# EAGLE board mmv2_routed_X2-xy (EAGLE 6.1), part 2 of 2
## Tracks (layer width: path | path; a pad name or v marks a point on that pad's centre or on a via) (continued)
GLC1P  (via drill 0.5) (continued)
  Top 0.2: R22.1 61.21,31.4 63.21,31.4 R21.1 63.31,31.4 67.31,31.4 | R19.1 73.31,29.5 73.21,29.5 71.31,31.4 R20.1 67.31,31.4 | R26.1 40.81,31.4 R25.1 46.91,31.4 | R23.1 53.01,31.5 51.01,31.5 R24.1 50.91,31.4 46.91,31.4 | 6.41,31.5 10.21,31.5 R32.1 10.31,31.4 12.31,31.4 R31.1 | 6.41,31.5 2.61,31.5 R33.1 | R34.1 25.51,43.2 21.31,43.2 20.41,44.1 D125.A | 21.51,31.4 22.51,31.4 R29.1 22.61,31.3 23.41,30.5 29.61,30.5 29.66,30.45 | 21.51,31.4 R30.1 | R27.1 32.71,31.4 30.71,31.4 R28.1 30.61,31.4 29.66,30.45 | 29.66,30.45 29.51,30.3 29.51,23.8 | 21.51,31.4 v21.51,32.7 | 6.41,23.8 6.41,31.5 | 46.91,23.8 46.91,31.4 | 67.31,23.8 67.31,31.4
  Top 1.676: D65.A D67.C D69.A D71.C 67.31,23.8 D75.C | D75.C D73.A | D75.C D77.A D79.C D83.C | D83.C D81.A | D83.C D85.A D87.C 46.91,23.8 D89.A D91.C D93.A D95.C D97.A D99.C D101.A 29.51,23.8 D103.C D105.A D107.C D109.A D111.C D113.A D115.C D117.A D119.C 6.41,23.8 D121.A D123.C
  Bottom 0.2: v21.51,32.7 21.51,39.9 20.61,40.8 D127.C | D95.C 39.31,22.6 39.31,7.3 38.11,6.1 JP21.2
  Bottom 1.676: D127.C D125.A
  pour Top: 79.51,33 79.51,0.5 0.51,0.5 0.51,33
GLCN
  Top 1.676: JP17.1 JP16.1 JP15.1 JP14.1 JP13.1 JP12.1 JP11.1 JP4.1 JP10.1 JP9.1 JP8.1 JP7.1 JP6.1 JP5.1 JP2.1 JP1.1
  Bottom 0.2: JP18.1 77.51,59.4 78.61,60.5 78.61,96.5 76.51,98.6 68.61,98.6 68.61,96.2 JP17.1
  pour Bottom (isolate 0.254): 79.51,99.5 79.51,55 64.51,55 64.01,95 9.51,95 9.51,99.5
GLCP
  Top 0.2: R10.1 38.01,69.5 35.91,69.5 R9.1 35.81,69.5 27.91,69.5 R8.1 27.81,69.6 25.71,69.6 R7.1 25.61,69.5 R6.1 15.61,69.5 R5.1 15.51,69.6 11.61,69.6 | R1.1 5.41,69.6 7.51,69.6 R2.1 7.61,69.6 11.61,69.6 | R14.1 58.31,69.6 56.21,69.6 R13.1 56.11,69.6 52.21,69.6 | R11.1 48.21,69.5 R12.1 48.31,69.6 52.21,69.6 | 72.51,69.5 R16.1 66.41,69.5 R15.1 | 72.51,69.5 76.41,69.5 R17.1 | R18.1 55.31,57.2 55.91,57.8 60.01,57.8 60.91,56.9 D63.C | 72.51,77.14 72.51,69.5 | 52.21,77.14 52.21,69.6 | 11.61,77.14 11.61,69.6
  Top 1.676: D1.A D3.C D5.A D7.C 11.61,77.14 D9.A D11.C D13.A D15.C D19.C | D19.C D17.A | D19.C D21.A D23.C D27.C | D27.C D25.A | D27.C D29.A D31.C D35.C | D35.C D33.A | D35.C D37.A D39.C 52.21,77.14 D43.C | D43.C D41.A | D43.C D45.A D47.C D51.C | D51.C D49.A | D59.C D57.A 72.51,77.14 D53.A | D53.A D55.C | D53.A D51.C
  Bottom 0.2: D47.C 61.91,76.2 61.91,60.7 61.31,60.1 D61.A | JP4.2 42.01,93.6 42.01,78.3 43.11,77.2 D33.A
  Bottom 1.676: D63.C D61.A
  pour Top (isolate 0.254): 79.51,99.5 79.51,68 0.51,68 0.51,99.5
GND  (via drill 0.5)  (1 unrouted)
  Top 0.2: OK1.3 2.61,65.8 3.51,66.7 9.21,66.7 10.11,65.8 OK2.3 10.21,65.7 OK3.3 12.71,65.8 13.61,66.7 19.41,66.7 20.31,65.8 OK4.3 20.41,65.7 22.81,65.7 OK5.3 22.91,65.8 23.81,66.7 29.51,66.7 30.41,65.8 OK6.3 30.51,65.7 33.01,65.7 OK7.3 33.11,65.8 34.01,66.7 39.71,66.7 40.61,65.8 OK8.3 40.71,65.7 43.11,65.7 OK9.3 | 25.41,35.3 OK27.3 25.41,35.2 24.51,34.3 18.71,34.3 17.81,35.2 OK28.3 17.71,35.3 15.31,35.3 OK29.3 15.21,35.2 14.31,34.3 8.61,34.3 7.71,35.2 OK30.3 7.61,35.3 5.11,35.3 OK31.3 | 34.21,53.8 U1.18 34.26,53.8 | X2.5 11.91,52.4 JP3.5 22.71,52.4 23.71,53.4 25.01,53.4 26.01,54.4 32.41,54.4 33.01,53.8 34.26,53.8 | OK10.3 53.31,65.7 OK11.3 | v47.81,53.6 47.41,53.8 45.71,53.8 U1.63 45.61,53.8 44.81,53.8 44.51,53.5 41.41,53.5 41.31,53.6 40.61,53.6 40.51,53.55 40.26,53.3 v38.51,53.3 | OK25.3 35.61,35.3 38.11,35.3 OK24.3 | v38.51,54.9 38.21,54.9 38.21,56.2 U1.12 | U1.31 34.31,47.3 35.71,47.3 v35.91,47.5 | OK19.3 66.11,35.3 68.51,35.3 OK18.3 68.61,35.2 69.51,34.3 75.31,34.3 76.21,35.2 OK17.3 | v70.61,46 70.31,45.7 68.21,45.7 X1.3 | OK14.3 71.21,65.7 73.61,65.7 OK15.3 | OK23.3 45.81,35.3 48.21,35.3 OK22.3 | v45.61,43.6 43.57,43.6 43.21,43.95 43.21,44.9 U1.47 | OK20.3 58.41,35.3 55.91,35.3 OK21.3 | OK12.3 61.01,65.7 OK13.3 | S1.4 56.71,49.7 60.41,49.7 61.51,48.6 C2.- 61.61,48.5 61.91,48.2 68.11,48.2 X1.5 | 34.26,53.8 35.01,53.8 35.71,54.5 v35.71,54.6
  Top 1.016: X2.3 2.62,55.01 1.91,54.3
  Bottom 0.2: X2.5 11.91,52.5 11.91,55 X2.3 11.91,55.1 12.91,56.1 12.91,65.5 OK3.3 | 25.41,35.3 25.11,35.6 25.11,46 23.61,47.5 23.61,51.5 22.71,52.4 JP3.5 | 25.41,35.3 OK27.3 | v47.81,53.6 49.51,56.3 49.51,56.8 OK16.3 49.61,56.9 50.51,57.8 50.51,65.4 OK10.3 | C5.2 38.91,56.3 38.91,55.3 v38.51,54.9 38.21,54.6 38.21,54.1 | C6.2 35.51,48.1 35.51,47.7 v35.91,47.5 36.31,47.1 36.31,36 35.61,35.3 OK25.3 35.61,35.2 35.71,35.1 35.71,32.8 37.01,31.5 44.41,31.5 45.41,32.5 45.41,34.9 45.71,35.2 OK23.3 45.71,35.3 45.61,35.4 v45.61,43.6 C9.2 | 38.21,53.3 38.21,52.5 34.71,49 C6.2 | 38.21,53.3 38.21,54.1 | 31.11,48 31.01,44.9 31.71,44.2 OK32.3 | 34.41,49.1 C6.2 | 38.21,53.3 v38.51,53.3 | C4.2 78.31,42.8 77.91,42.4 77.91,37 76.21,35.3 OK17.3 | v70.61,46 72.31,46 IC1.1 | OK14.3 71.11,65.7 69.61,64.2 69.61,54.1 C3.2 69.51,54 69.21,53.7 69.21,49.3 68.21,48.3 X1.5 68.21,48.2 68.21,45.7 X1.3 68.11,45.6 67.11,44.6 67.11,36.3 66.11,35.3 OK19.3 | C10.2 54.81,42.7 54.81,38.9 | 54.81,38.9 54.81,36.3 54.86,36.25 | 54.86,36.25 55.81,35.3 OK21.3 | SJ1.1 57.61,52.3 57.11,51.8 57.11,50.2 56.71,49.8 S1.4 57.11,50.1 57.11,47.1 57.61,46.6 SJ4.1 | SJ4.1 59.61,46.6 61.61,48.6 C1.- 61.71,48.7 62.31,49.3 62.31,64.5 OK13.3 | SJ4.1 57.51,46.6 57.51,44.1 56.71,43.3 S1.3 56.61,43.2 56.61,38.9 54.81,38.9 | OK22.3 48.31,35.2 49.51,34 54.81,34 54.81,36.2 54.86,36.25 | 38.21,54.1 37.11,54.1 36.01,55.2 36.01,57.2 36.51,57.7 36.51,67 34.61,67 33.11,65.8 OK7.3 | OK26.3 25.48,35.23 25.41,35.3
  other vias: 27.81,54.4
  pour Bottom: 0.51,70.5 0.51,47 20.01,47 20.51,25.5 83.01,25.5 79.51,54 63.51,54 63.01,54.5 63.01,70.5
GND1  (via drill 0.61)
  Top 0.508: C11.- 152.22,75.7 150.82,74.3 150.82,71.6 C12.- 150.82,71.3 150.92,71.2 150.92,62.7 150.77,62.55 | JP39.1 156.82,59.3 156.12,59.3 153.12,62.3 R74.1 152.82,62.3 151.02,62.3 150.77,62.55 | 150.77,62.55 148.52,64.8 J1.2 | C7.2 95.02,78.9 95.42,79.3 95.42,81.6 C13.- | C7.2 94.72,78.8 92.02,78.8 C8.2 91.82,79 91.82,81.6 JP38.3 | 96.32,76.4 96.32,77.7 95.22,78.8 C7.2 | 96.32,76.4 96.32,69.1 98.42,67 IC4.5 | v142.92,75.6 142.92,94 146.02,97.1 JP37.1 | v103.92,76.4 96.32,76.4
  Bottom 0.508: R75.1 142.72,97.1 146.02,97.1 JP37.1 | IC2.5 133.52,79 136.42,79 C16.2 136.52,78.8 139.22,76.1 139.22,75.3 | 147.97,74.25 146.72,75.5 IC3.GND | 147.97,74.25 148.12,74.1 148.42,74.1 148.92,73.6 C14.2 | C15.2 144.42,73.6 144.92,74.1 147.82,74.1 147.97,74.25 | 139.22,75.3 139.22,75.2 142.42,75.2 | 142.42,75.2 144.12,73.5 C15.2 | v142.92,75.6 142.62,75.3 142.42,75.2 | v103.92,76.4 131.22,76.4 132.32,75.3 139.22,75.3 | J1.2 148.42,64.9 147.22,66.1 144.12,66.1 143.32,66.9 143.32,70.6 143.72,71 143.72,73.3 144.02,73.3 C15.2
  pour Top: 159.02,53.5 88.52,53.5 88.52,99.5 159.02,99.5
GND2  (via drill 0.61)
  Top 0.508: C19.- 152.22,23.7 150.82,22.3 150.82,19.6 C20.- 150.82,19.3 150.92,19.2 150.92,10.7 150.77,10.55 | JP42.1 156.82,7.3 156.12,7.3 153.12,10.3 R84.1 152.82,10.3 151.02,10.3 150.77,10.55 | 150.77,10.55 148.52,12.8 J2.2 | C17.2 95.02,26.9 95.42,27.3 95.42,29.6 C21.- | C17.2 94.72,26.8 92.02,26.8 C18.2 91.82,27 91.82,29.6 JP41.3 | 96.32,24.4 96.32,25.7 95.22,26.8 C17.2 | 96.32,24.4 96.32,17.1 98.42,15 IC7.5 | v142.92,23.6 142.92,42 146.02,45.1 JP40.1 | v103.92,24.4 96.32,24.4
  Bottom 0.508: R85.1 142.72,45.1 146.02,45.1 JP40.1 | IC5.5 133.52,27 136.42,27 C24.2 136.52,26.8 139.22,24.1 139.22,23.3 | 147.97,22.25 146.72,23.5 IC6.GND | 147.97,22.25 148.12,22.1 148.42,22.1 148.92,21.6 C22.2 | C23.2 144.42,21.6 144.92,22.1 147.82,22.1 147.97,22.25 | 139.22,23.3 139.22,23.2 142.42,23.2 | 142.42,23.2 144.12,21.5 C23.2 | v142.92,23.6 142.62,23.3 142.42,23.2 | v103.92,24.4 131.22,24.4 132.32,23.3 139.22,23.3 | J2.2 148.42,12.9 147.22,14.1 144.12,14.1 143.32,14.9 143.32,18.6 143.72,19 143.72,21.3 144.02,21.3 C23.2
  pour Top: 159.02,1.5 88.52,1.5 88.52,47.5 159.02,47.5
I2C_SCL  (via drill 0.5)
  Top 0.2: v39.31,75.1 38.91,75.5 v24.51,75.5 | U1.61 45.61,52.8 44.61,52.8 44.41,53 41.21,53 v41.01,52.8
  Bottom 0.2: v41.01,52.8 41.41,53.2 41.41,62.4 39.31,64.5 v39.31,75.1 | v24.51,75.5 23.81,74.8 23.81,72.7 21.91,70.8 21.91,64.1 | 21.91,64.1 21.91,59.5 22.61,58.8 22.61,57.5 JP3.1 | R67.1 18.31,58.7 18.31,60.5 21.91,64.1
I2C_SDA  (via drill 0.5)
  Top 0.2: v50.81,53.3 50.31,52.8 47.01,52.8 46.51,53.3 45.71,53.3 U1.62 | v50.21,68.3 50.01,68.5 24.71,68.5 24.31,68.9 23.21,68.9 v23.01,68.7
  Bottom 0.2: v50.81,53.3 51.21,53.7 51.21,63.6 51.81,64.2 51.81,66.7 v50.21,68.3 | v23.01,68.7 23.51,68.7 23.71,68.9 24.81,68.9 24.81,67.7 24.31,67.2 24.31,58.3 25.11,57.5 JP3.2 27.1,59.4 R68.1
MES  (via drill 0.61)
  Top 0.254: v90.62,77.1 91.92,77.1 C8.1 91.92,77 95.62,73.3 95.62,64.8 v100.62,59.8 | v129.72,59 130.32,59.6 130.32,63.6 135.82,69.1 v135.82,85.6
  Bottom 0.254: v90.62,77.1 91.82,77.1 R77.2 | v100.62,59.8 101.42,59 v129.72,59 | v135.82,85.6 139.32,89.1 141.02,89.1 IC2.18
MES1  (via drill 0.61)
  Top 0.254: v90.62,25.1 91.92,25.1 C18.1 91.92,25 95.62,21.3 95.62,12.8 v100.62,7.8 | v129.72,7 130.32,7.6 130.32,11.6 135.82,17.1 v135.82,33.6
  Bottom 0.254: v90.62,25.1 91.82,25.1 R87.2 | v100.62,7.8 101.42,7 v129.72,7 | v135.82,33.6 139.32,37.1 141.02,37.1 IC5.18
N$1  (via drill 0.5)
  Top 0.2: v55.51,54.2 53.61,52.3 45.71,52.3 U1.60
  Bottom 0.2: 55.51,53.6 v55.51,54.2 | R65.1 55.51,53.6 | 55.51,53.6 56.11,53.6 56.11,52.3 SJ1.2
N$2
  Bottom 1.676: D3.A D4.C
N$3
  Bottom 1.676: D1.C D2.A
N$4
  Top 1.676: D4.A D2.C
  Bottom 0.2: OK1.2 2.61,73.4 3.91,74.7 3.91,88.6 4.91,89.6 D4.A
  Bottom 0.61: 8.01,91.7 7.81,91.7 7.41,91.3 7.11,91.3 6.61,90.8 6.05,90.8 D4.A
  Bottom 1.016: JP1.2 9.96,93.65 8.01,91.7
N$5
  Top 0.2: R1.2 5.31,71.5 5.31,73.3 5.11,73.3 OK1.1
N$6
  Bottom 1.676: D19.A D20.C
N$7
  Bottom 1.676: D7.A D8.C
N$8
  Bottom 1.676: D5.C D6.A
N$9
  Top 1.676: D6.C D8.A
  Bottom 0.2: OK2.2 10.11,73.4 9.01,74.5 9.01,88.5 9.91,89.4 D8.A
  Bottom 1.016: JP2.2 13.31,91.7 12.03,91.7 D8.A
N$10
  Top 0.2: R2.2 7.61,71.5 7.61,73.3 OK2.1
N$11
  Bottom 1.676: D11.A D12.C
N$12
  Top 0.2: LED17.A 73.11,39.2 74.01,38.3 74.61,38.3 R49.1
N$13  (via drill 0.61)
  Top 0.254: v119.72,62.5 120.12,62.1 120.12,55.4 120.82,54.7 140.12,54.7 v140.12,55.6
  Bottom 0.254: v119.72,62.5 117.12,65.1 100.32,65.1 100.32,67.6 98.52,69.4 IC4.6 | v140.12,55.6 140.22,55.7 142.62,55.7 144.22,57.3 144.22,61.8 143.02,61.8 142.42,62.4 142.42,63.8 144.82,63.8 145.82,64.8 J1.4
N$14
  Top 0.2: R3.1 4.91,62.7 5.81,61.8 LED1.A
N$15  (via drill 0.5)
  Top 0.2: v47.41,55.9 47.71,55.6 v52.41,55.6 | U1.7 40.71,56.3 40.71,58.5 41.21,59 46.91,59 v47.41,58.5
  Bottom 0.2: v47.41,55.9 v47.41,58.5 | v52.41,55.6 52.21,55.4 52.21,49.8 S1.2 52.21,49.7 52.21,49.4 R66.1 54.01,47.6 54.01,45.5 C10.1 52.91,44.4 52.91,44 52.21,43.3 S1.1
N$16
  Top 0.2: R4.1 7.71,62.7 LED2.A
N$17
  Bottom 1.676: D9.C D10.A
N$18  (via drill 0.5)
  Top 0.2: v16.01,75.6 14.91,75.6 12.71,73.4 OK3.2
  Top 1.676: D12.A D10.C
  Bottom 0.2: v16.01,75.6 16.41,76 16.41,90.3 16.06,90.65
  Bottom 1.016: JP5.2 16.06,90.65 D12.A
N$19
  Top 0.2: R5.2 15.51,71.5 15.51,73.3 15.31,73.3 OK3.1
N$20
  Bottom 1.676: D17.C D18.A
N$21
  Bottom 1.676: D15.A D16.C
N$22
  Bottom 1.676: D13.C D14.A
N$23
  Top 1.676: D16.A D14.C
  Bottom 0.2: OK4.2 20.41,73.4 21.51,74.5 21.51,88.3 20.71,89.1 D16.A
  Bottom 1.676: JP6.2 20.33,91.11 D16.A
N$24
  Top 0.2: R6.2 17.71,71.4 17.71,73.3 OK4.1
N$25
  Top 1.676: D20.A D18.C
  Bottom 0.2: OK5.2 22.91,73.4 23.41,73.9 23.41,76.1 24.01,76.7 24.01,88.3 22.91,89.4 22.91,89.8 D18.C
  Bottom 1.676: JP7.2 25.41,92.38 D20.A
N$26
  Top 0.2: R7.2 25.61,71.5 25.61,73.3 25.41,73.3 OK5.1
N$27
  Bottom 1.676: D23.A D24.C
N$28
  Bottom 1.676: D21.C D22.A
N$29
  Top 1.676: D24.A D22.C
  Bottom 0.2: OK6.2 30.41,73.4 29.31,74.5 29.31,88.3 30.11,89.1 D24.A
  Bottom 1.676: JP8.2 D24.A
N$30
  Top 0.2: R8.2 27.91,71.5 27.91,73.3 OK6.1
N$31
  Bottom 1.676: D27.A D28.C
N$32
  Bottom 1.676: D25.C D26.A
N$33
  Top 1.676: D28.A D26.C
  Bottom 0.2: OK7.2 33.11,73.4 34.21,74.5 34.21,88.3 33.41,89.1 D26.C
  Bottom 1.676: JP9.2 33.03,92.38 D26.C
N$34
  Top 0.2: R9.2 35.81,71.5 35.81,73.3 35.61,73.3 OK7.1
N$35
  Bottom 1.676: D31.A D32.C
N$36
  Bottom 1.676: D29.C D30.A
N$37
  Top 1.676: D32.A D30.C
  Bottom 0.2: OK8.2 40.61,73.4 40.11,73.9 40.11,76.1 39.51,76.7 39.51,88.1 40.61,89.2 40.61,89.8 D32.A
  Bottom 1.676: JP10.2 D30.C
N$38
  Top 0.2: OK8.1 38.11,71.4 R10.2
N$39
  Bottom 1.676: D35.A D36.C
N$40
  Bottom 1.676: D33.C D34.A
N$41
  Top 1.676: D34.C D36.A
  Bottom 0.2: OK9.2 43.21,73.4 44.51,74.7 44.51,88.5 45.21,89.2 D36.A
  Bottom 1.676: JP11.2 D36.A
N$42
  Top 0.2: R11.2 46.01,71.4 46.01,73.3 45.81,73.3 OK9.1
N$43
  Bottom 1.676: D39.A D40.C
N$44
  Bottom 1.676: D37.C D38.A
N$45
  Top 1.676: D40.A D38.C
  Bottom 0.2: OK10.2 50.81,73.4 52.01,74.6 52.01,88.3 51.21,89.1 D40.A
  Bottom 1.676: JP12.2 50.81,92.38 D40.A
N$46
  Top 0.2: R12.2 48.21,71.5 48.21,73.3 OK10.1
N$47
  Bottom 1.676: D43.A D44.C
N$48
  Bottom 1.676: D41.C D42.A
N$49
  Top 1.676: D42.C D44.A
  Bottom 0.2: OK11.2 53.41,73.4 54.51,74.5 54.51,88.3 53.71,89.1 D42.C
  Bottom 1.676: JP13.2 D42.C
N$50
  Top 0.2: R13.2 56.11,71.5 56.11,73.3 55.91,73.3 OK11.1
N$51
  Bottom 1.676: D48.C D47.A
N$52
  Bottom 1.676: D45.C D46.A
N$53
  Top 1.676: D48.A D46.C
  Bottom 0.2: OK12.2 60.91,73.4 59.61,74.7 59.61,88.3 58.81,89.1 D46.C
  Bottom 1.676: JP14.2 58.43,92.38 D46.C
N$54
  Top 0.2: R14.2 58.41,71.5 58.41,73.3 OK12.1
N$55
  Bottom 1.676: D52.C D51.A
N$56
  Bottom 1.676: D49.C D50.A
N$57
  Top 1.676: D50.C D52.A
  Bottom 0.2: OK13.2 63.51,73.4 64.71,74.6 64.71,88.3 63.91,89.1 D50.C
  Bottom 1.676: JP15.2 63.51,91.11 D50.C
N$58
  Top 0.2: R15.2 66.31,71.5 66.31,73.3 66.11,73.3 OK13.1
N$59
  Bottom 1.676: D55.A D56.C
N$60
  Bottom 1.676: D53.C D54.A
N$61
  Top 1.676: D54.C D56.A
  Bottom 0.2: OK14.2 71.21,73.4 72.31,74.5 72.31,88.7 71.21,89.8 D56.A
  Bottom 1.016: JP16.2 D54.C
N$62
  Top 0.2: R16.2 68.51,71.4 68.51,73.3 OK14.1
N$63
  Bottom 1.676: D59.A D60.C
N$64
  Bottom 1.676: D57.C D58.A
N$65
  Top 1.676: D60.A D58.C
  Bottom 0.2: OK15.2 73.71,73.4 74.81,74.5 74.81,88.5 73.91,89.4 D58.C
  Bottom 1.016: JP17.2 69.86,93.65 D58.C
N$66
  Top 0.2: R17.2 76.41,71.5 76.41,73.3 76.21,73.3 OK15.1
N$67
  Top 1.676: D63.A D64.C
N$68
  Top 1.676: D61.C D62.A
N$69
  Top 0.2: OK16.2 57.21,56.8 58.41,55.6 72.31,55.6 73.01,56.3 D64.A
  Top 1.676: JP18.2 77.45,56.82 D64.A
  Bottom 1.676: D62.C D64.A
N$70
  Top 0.2: R18.2 55.31,59.1 55.51,59.3 57.11,59.3 OK16.1
N$71
  Bottom 1.676: D68.C D67.A
N$72
  Bottom 1.676: D66.A D65.C
N$73
  Top 1.676: D66.C D68.A
  Bottom 0.2: OK17.2 74.81,26.2 74.81,11.2 73.91,10.3 D68.A
  Bottom 1.016: JP19.2 69.86,6.02 D68.A
N$74
  Top 0.2: R19.2 73.41,31.3 74.21,30.5 74.31,30.5 74.51,30.3 74.51,27.7 73.71,27.7 OK17.1
N$75
  Bottom 1.676: D72.C D71.A
N$76
  Bottom 1.676: D70.A D69.C
N$77
  Top 1.676: D70.C D72.A
  Bottom 0.2: OK18.2 68.51,27.6 67.41,26.5 67.41,9.3 67.74,8.97
  Bottom 1.016: JP20.2 67.74,8.97 D72.A
N$78
  Top 0.2: R20.2 71.21,29.5 71.21,27.7 OK18.1
N$79
  Bottom 1.676: D75.A D76.C
N$80
  Bottom 1.676: D74.A D73.C
N$81
  Top 1.676: D74.C D76.A
  Bottom 0.2: OK19.2 66.01,27.6 64.71,26.3 64.71,11.2 64.01,10.5 D76.A
  Bottom 1.676: JP22.2 63.51,8.56 D76.A
N$82
  Top 0.2: R21.2 63.31,29.5 63.31,27.7 63.51,27.7 OK19.1
N$83
  Bottom 1.676: D80.C D79.A
N$84
  Bottom 1.676: D78.A D77.C
N$85
  Top 1.676: D78.C D80.A
  Bottom 0.2: OK20.2 58.51,27.6 59.61,26.5 59.61,11.2 58.91,10.5 D80.A
  Bottom 1.676: JP23.2 58.43,7.29 D80.A
N$86
  Top 0.2: R22.2 61.11,29.4 61.11,27.7 61.01,27.7 OK20.1
N$87  (via drill 0.61)
  Top 0.254: v110.02,71.5 112.12,69.4 v112.12,55.8
  Bottom 0.254: v110.02,71.5 99.02,71.5 98.52,72 IC4.7 | v112.12,55.8 113.22,54.7 142.92,54.7 153.32,65.1 153.32,66.3 148.22,66.3 147.22,67.3 J1.3
N$88
  Bottom 1.676: D84.C D83.A
N$89
  Bottom 1.676: D82.A D81.C
N$90
  Top 1.676: D82.C D84.A
  Bottom 0.2: OK21.2 55.81,27.6 54.51,26.3 54.51,11.2 53.81,10.5 D84.A
  Bottom 1.676: JP24.2 D84.A
N$91
  Top 0.2: R23.2 53.11,29.5 53.11,27.7 53.31,27.7 OK21.1
N$92
  Bottom 1.676: D88.C D87.A
N$93
  Bottom 1.676: D86.A D85.C
N$94
  Top 1.676: D88.A D86.C
  Bottom 0.2: OK22.2 48.21,27.6 47.11,26.5 47.11,11 48.21,9.9 D88.A
  Bottom 1.676: JP25.2 50.81,7.29 D86.C
N$95
  Top 0.2: R24.2 50.91,29.5 50.91,27.7 50.81,27.7 OK22.1
N$96
  Bottom 1.676: D91.A D92.C
N$97
  Bottom 1.676: D90.A D89.C
N$98
  Top 1.676: D92.A D90.C
  Bottom 0.2: OK23.2 45.71,27.6 44.51,26.4 44.51,11.5 45.41,10.6 D90.C
  Bottom 1.676: JP26.2 D90.C
N$99
  Top 0.2: R25.2 42.91,29.5 42.91,27.7 43.11,27.7 OK23.1
N$100
  Bottom 1.676: D95.A D96.C
N$101
  Bottom 1.676: D93.C D94.A
N$102
  Top 1.676: D94.C D96.A
  Bottom 0.2: OK24.2 36.91,26.4 36.91,11.1 38.11,9.9 D96.A
  Bottom 1.676: JP27.2 40.65,7.29 D94.C
N$103
  Top 0.2: R26.2 40.71,29.4 40.71,27.7 OK24.1
N$104
  Bottom 1.676: D100.C D99.A
N$105
  Bottom 1.676: D98.A D97.C
N$106
  Top 1.676: D98.C D100.A
  Bottom 0.2: OK25.2 35.51,27.6 34.21,26.3 34.21,11.2 33.51,10.5 D100.A
  Bottom 1.676: JP28.2 33.03,7.29 D100.A
N$107
  Top 0.2: R27.2 32.81,29.5 32.81,27.7 33.01,27.7 OK25.1
N$108
  Bottom 1.676: D103.A D104.C
N$109
  Bottom 1.676: D102.A D101.C
N$110
  Top 1.676: D102.C D104.A
  Bottom 0.2: OK26.2 28.01,27.6 29.31,26.3 29.31,11.2 30.01,10.5 D102.C
  Bottom 1.676: JP29.2 D102.C
N$111
  Top 0.2: R28.2 30.61,29.5 30.61,27.7 30.51,27.7 OK26.1
N$112
  Bottom 1.676: D107.A D108.C
N$113
  Bottom 1.676: D105.C D106.A
N$114
  Top 1.676: D106.C D108.A
  Bottom 0.2: OK27.2 26.61,26.4 26.61,11.2 25.91,10.5 D106.C
  Bottom 1.676: JP30.2 25.41,7.29 D106.C
N$115
  Top 0.2: R29.2 22.61,29.4 22.61,27.7 22.81,27.7 OK27.1
N$116
  Bottom 1.676: D111.A D112.C
N$117
  Bottom 1.676: D109.C D110.A
N$118
  Top 1.676: D110.C D112.A
  Bottom 0.2: OK28.2 17.81,27.6 19.11,26.3 19.11,11.5 20.01,10.6 D110.C
  Bottom 1.676: JP31.2 20.33,8.56 D110.C
N$119
  Top 0.2: R30.2 20.41,29.5 20.41,27.7 OK28.1
N$120
  Bottom 1.676: D115.A D116.C
N$121
  Bottom 1.676: D113.C D114.A
N$122
  Top 1.676: D116.A D114.C
  Bottom 0.2: OK29.2 15.31,27.6 16.41,26.5 16.41,9.4 16.06,9.05 | 15.31,9.8 D114.C 15.11,9.9
  Bottom 1.016: JP32.2 19.06,6.05 16.06,9.05 15.31,9.8 15.21,9.9 15.11,9.9 15.01,9.8
N$123
  Top 0.2: R31.2 12.41,29.5 12.41,27.7 12.71,27.7 OK29.1
N$124
  Bottom 1.676: D119.A D120.C
N$125
  Bottom 1.676: D117.C D118.A
N$126
  Top 1.676: D120.A D118.C
  Bottom 0.2: OK30.2 7.71,27.6 9.01,26.3 9.01,11.3 10.01,10.3 D118.C
  Bottom 1.016: JP33.2 13.17,8.1 11.91,8.1 D118.C
N$127
  Top 0.2: R32.2 10.21,29.5 10.21,27.7 OK30.1
N$128
  Bottom 1.676: D123.A D124.C
N$129
  Bottom 1.676: D121.C D122.A
N$130
  Top 1.676: D124.A D122.C
  Bottom 0.2: 6.31,8.8 6.31,26.4 5.11,27.6 OK31.2
  Bottom 0.61: 7.91,8.1 arc-50 6.41,8.8 6.31,8.8 6.12,8.8 D122.C
  Bottom 1.016: JP34.2 9.36,8.1 7.91,8.1
N$131
  Top 0.2: R33.2 2.61,29.5 2.61,27.7 OK31.1
N$132
  Top 1.676: D127.A D128.C
N$133
  Top 1.676: D125.C D126.A
N$134
  Top 0.2: OK32.2 24.11,44.2 23.01,45.3 8.81,45.3 D126.C 7.61,44.1 | 3.91,44.1 JP35.2
  Top 1.27: 3.91,44.1 3.91,44.12 D126.C
  Bottom 1.676: D126.C D128.A
N$135
  Top 0.2: R34.2 25.81,41.6 24.21,41.6 OK32.1
N$136  (via drill 0.61)
  Top 0.254: v119.72,10.5 120.12,10.1 120.12,3.4 120.82,2.7 140.12,2.7 v140.12,3.6
  Bottom 0.254: v119.72,10.5 117.12,13.1 100.32,13.1 100.32,15.6 98.52,17.4 IC7.6 | v140.12,3.6 140.22,3.7 142.62,3.7 144.22,5.3 144.22,9.8 143.02,9.8 142.42,10.4 142.42,11.8 144.82,11.8 145.82,12.8 J2.4
N$137
  Top 0.2: R35.1 15.11,62.7 16.01,61.8 LED3.A
N$138  (via drill 0.61)
  Top 0.254: v110.02,19.5 112.12,17.4 v112.12,3.8
  Bottom 0.254: v110.02,19.5 99.02,19.5 98.52,20 IC7.7 | v112.12,3.8 113.22,2.7 142.92,2.7 153.32,13.1 153.32,14.3 148.22,14.3 147.22,15.3 J2.3
N$139
  Top 0.2: R36.1 17.91,62.7 17.01,61.8 LED4.A
N$141
  Top 0.2: R37.1 25.31,62.7 26.21,61.8 LED5.A
N$143
  Top 0.2: R38.1 28.11,62.7 27.21,61.8 LED6.A
N$145
  Top 0.2: R39.1 35.41,62.7 LED7.A
N$147
  Top 0.2: R40.1 38.11,62.7 37.31,61.9 LED8.A
N$149
  Top 0.2: R41.1 45.61,62.7 46.51,61.8 LED9.A
N$151
  Top 0.2: R42.1 48.41,62.7 47.51,61.8 LED10.A
N$153
  Top 0.2: R43.1 55.71,62.7 56.61,61.8 LED11.A
N$155
  Top 0.2: R44.1 58.51,62.6 LED12.A
N$157
  Top 0.2: R45.1 66.01,62.6 66.81,61.8 LED13.A
N$159
  Top 0.2: R46.1 68.61,62.6 67.81,61.8 LED14.A
N$161
  Top 0.2: R47.1 76.21,62.6 77.01,61.8 LED15.A
N$163
  Top 0.2: LED16.A 51.01,57.4 52.61,59 52.91,59 R48.1
N$164
  Top 0.2: LED18.A 71.81,39.2 70.91,38.3 70.31,38.3 R50.1
N$165
  Top 0.2: LED19.A 62.71,39.2 63.61,38.3 64.21,38.3 R51.1
N$166
  Top 0.2: LED20.A 61.51,39.2 60.61,38.3 60.11,38.3 R52.1
N$167
  Top 0.2: LED21.A 52.61,39.2 53.51,38.3 54.01,38.3 R53.1
N$168
  Top 0.2: LED22.A 51.51,39.1 50.71,38.3 50.01,38.3 R54.1
N$169
  Top 0.2: LED23.A 42.51,39.2 43.41,38.3 44.01,38.3 R55.1
N$170
  Top 0.2: LED24.A 41.41,39.2 40.51,38.3 39.91,38.3 R56.1
N$171
  Top 0.2: LED25.A 32.41,39.3 33.41,38.3 33.81,38.3 R57.1
N$172
  Top 0.2: LED26.A 31.21,39.3 30.21,38.3 29.81,38.3 R58.1
N$173
  Top 0.2: LED27.A 22.21,39.2 23.11,38.3 23.71,38.3 R59.1
N$174
  Top 0.2: LED28.A 21.11,39.2 20.21,38.3 19.61,38.3 R60.1
N$175
  Top 0.2: LED29.A 12.11,39.2 13.01,38.3 13.51,38.3 R61.1
N$176
  Top 0.2: LED30.A 10.91,39.2 10.01,38.3 9.51,38.3 R62.1
N$177
  Top 0.2: LED31.A 2.01,39.2 2.91,38.3 3.41,38.3 R63.1
N$178
  Top 0.2: R64.1 30.21,43.7 30.31,43.6 LED32.A
POT
  Top 0.254: C13.+ 92.32,84.8 JP38.2
  Bottom 0.254: JP38.2 89.22,84.8 89.22,87.8 89.92,88.5 93.22,88.5 98.52,93.8 105.52,93.8 105.92,93.4 112.92,93.4 113.02,93.3 115.72,93.3 118.22,95.8 119.52,95.8 121.52,93.8 128.82,93.8 133.42,89.2 IC2.1
POT1
  Top 0.254: C21.+ 92.32,32.8 JP41.2
  Bottom 0.254: JP41.2 89.22,32.8 89.22,35.8 89.92,36.5 93.22,36.5 98.52,41.8 105.52,41.8 105.92,41.4 112.92,41.4 113.02,41.3 115.72,41.3 118.22,43.8 119.52,43.8 121.52,41.8 128.82,41.8 133.42,37.2 IC5.1
POTH
  Bottom 0.254: R78.2 93.72,87.3 91.22,87.3 JP38.1
POTH1
  Bottom 0.254: R88.2 93.72,35.3 91.22,35.3 JP41.1
PWM  (via drill 0.61)
  Top 0.254: v126.42,81.1 131.72,81.1 131.72,70.6 133.42,68.9 IC2.9
  Bottom 0.254: v126.42,81.1 101.12,81.1 97.12,77.1 R76.1
PWM1  (via drill 0.61)
  Top 0.254: v126.42,29.1 131.72,29.1 131.72,18.6 133.42,16.9 IC5.9
  Bottom 0.254: v126.42,29.1 101.12,29.1 97.12,25.1 R86.1
ROW1  (via drill 0.61)
  Top 0.254: S2.1 128.82,96.6 128.82,90.2 S2.2 128.82,90.1 128.82,85.5 S3.1 128.92,85.4 131.72,82.6 135.22,82.6 135.22,78.1 v134.92,77.8 | S3.2 128.82,78.9 128.82,74.4 S4.1 128.82,74.2 128.82,67.9 S4.2 128.82,67.8 128.82,63.2 S5.1 128.82,63.1 128.82,56.7 S5.2
  Bottom 0.254: D129.1 127.42,92.6 127.42,90.2 128.82,90.2 S2.2 | v134.92,77.8 134.82,77.9 129.92,77.9 128.92,78.9 S3.2
ROW2
  Top 0.254: S6.1 121.22,96.6 121.22,90.2 S6.2 121.22,90.1 121.22,85.5 S7.1 121.22,85.4 121.22,79 S7.2 121.22,78.9 121.22,74.4 S8.1 121.22,74.2 121.22,67.9 S8.2 121.22,67.8 121.22,63.2 S9.1 121.22,63.1 121.22,56.7 S9.2
  Bottom 0.254: D130.1 119.92,92.4 119.92,90.2 121.22,90.2 S6.2
ROW3
  Top 0.254: S10.1 113.62,96.6 113.62,90.2 S10.2 113.62,90 113.62,85.5 S11.1 113.62,85.4 113.62,79 S11.2 113.62,78.9 113.62,74.4 S12.1 113.62,74.2 113.62,67.9 S12.2 113.62,67.8 113.62,63.2 S13.1 113.62,63.1 113.62,56.7 S13.2
  Bottom 0.254: D131.1 112.42,92.2 112.42,90.2 113.62,90.2 S10.2
ROW4
  Top 0.254: S14.1 106.02,96.6 106.02,90.2 S14.2 106.02,90 106.02,85.5 S15.1 106.02,85.4 106.02,79 S15.2 106.02,78.9 106.02,74.4 S16.1 106.02,74.2 106.02,67.9 S16.2 106.02,63.2 S17.1 106.02,63.1 106.02,56.7 S17.2
  Bottom 0.254: D132.1 104.92,90.2 105.92,90.2 S14.2
ROW5  (via drill 0.61)
  Top 0.254: S18.1 128.82,44.6 128.82,38.2 S18.2 128.82,38.1 128.82,33.5 S19.1 128.92,33.4 131.72,30.6 135.22,30.6 135.22,26.1 v134.92,25.8 | S19.2 128.82,26.9 128.82,22.4 S20.1 128.82,22.2 128.82,15.9 S20.2 128.82,15.8 128.82,11.2 S21.1 128.82,11.1 128.82,4.7 S21.2
  Bottom 0.254: D134.1 127.42,40.6 127.42,38.2 128.82,38.2 S18.2 | v134.92,25.8 134.82,25.9 129.92,25.9 128.92,26.9 S19.2
ROW6
  Top 0.254: S22.1 121.22,44.6 121.22,38.2 S22.2 121.22,38.1 121.22,33.5 S23.1 121.22,33.4 121.22,27 S23.2 121.22,26.9 121.22,22.4 S24.1 121.22,22.2 121.22,15.9 S24.2 121.22,15.8 121.22,11.2 S25.1 121.22,11.1 121.22,4.7 S25.2
  Bottom 0.254: D135.1 119.92,40.4 119.92,38.2 121.22,38.2 S22.2
ROW7
  Top 0.254: S26.1 113.62,44.6 113.62,38.2 S26.2 113.62,38 113.62,33.5 S27.1 113.62,33.4 113.62,27 S27.2 113.62,26.9 113.62,22.4 S28.1 113.62,22.2 113.62,15.9 S28.2 113.62,15.8 113.62,11.2 S29.1 113.62,11.1 113.62,4.7 S29.2
  Bottom 0.254: D136.1 112.42,40.2 112.42,38.2 113.62,38.2 S26.2
ROW8
  Top 0.254: S30.1 106.02,44.6 106.02,38.2 S30.2 106.02,38 106.02,33.5 S31.1 106.02,33.4 106.02,27 S31.2 106.02,26.9 106.02,22.4 S32.1 106.02,22.2 106.02,15.9 S32.2 106.02,11.2 S33.1 106.02,11.1 106.02,4.7 S33.2
  Bottom 0.254: D137.1 104.92,38.2 105.92,38.2 S30.2
RS  (via drill 0.61)
  Top 0.254: v145.32,80.5 144.92,80.9 144.92,89.9 145.92,90.9 147.42,90.9 147.42,93.4 148.52,94.5 JP37.4
  Bottom 0.254: IC2.16 141.12,84.2 145.22,88.3 149.02,88.3 150.02,89.3 150.02,94.5 148.62,94.5 JP37.4 | v145.32,80.5 152.12,80.5 152.12,71.6 156.82,66.9 JP39.4
RS1  (via drill 0.61)
  Top 0.254: v145.32,28.5 144.92,28.9 144.92,37.9 145.92,38.9 147.42,38.9 147.42,41.4 148.52,42.5 JP40.4
  Bottom 0.254: IC5.16 141.12,32.2 145.22,36.3 149.02,36.3 150.02,37.3 150.02,42.5 148.62,42.5 JP40.4 | v145.32,28.5 152.12,28.5 152.12,19.6 156.82,14.9 JP42.4
RS232_RX  (via drill 0.5)
  Top 0.2: v28.11,48.1 30.01,48.1 30.31,47.8 34.21,47.8 U1.30
  Bottom 0.2: v28.11,48.1 27.71,48.5 27.71,50.6 26.91,51.4 24.21,51.4 24.21,54 25.11,54.9 JP3.4
RS232_TX  (via drill 0.5)
  Top 0.2: v40.41,67.7 40.01,68.1 v24.01,68.1 | U1.29 37.89,48.28 38.61,49 38.61,49.2 v39.11,49.7
  Bottom 0.2: v40.41,67.7 41.81,66.3 41.81,52.4 v39.11,49.7 | v24.01,68.1 23.81,67.9 23.81,56.1 22.71,55 JP3.3
RWN  (via drill 0.61)
  Top 0.254: v153.12,79.8 154.02,80.7 154.02,90.7 149.02,95.7 147.22,95.7 147.22,93.9 146.12,92.8 146.12,92.1 JP37.5
  Bottom 0.254: R75.2 142.72,95.4 146.02,92.1 JP37.5 | v153.12,79.8 153.12,71.6 153.72,71 155.32,71 156.82,69.5 JP39.5
RWN1  (via drill 0.61)
  Top 0.254: v153.12,27.8 154.02,28.7 154.02,38.7 149.02,43.7 147.22,43.7 147.22,41.9 146.12,40.8 146.12,40.1 JP40.5
  Bottom 0.254: R85.2 142.72,43.4 146.02,40.1 JP40.5 | v153.12,27.8 153.12,19.6 153.72,19 155.32,19 156.82,17.5 JP42.5
RX  (via drill 0.61)
  Top 0.254: v130.82,73.3 129.72,72.2 v129.72,71.3 | v94.32,71 90.82,74.5 IC4.1
  Bottom 0.254: v130.82,73.3 132.82,73.3 133.42,73.9 IC2.7 | v129.72,71.3 128.12,69.7 100.32,69.7 99.02,71 v94.32,71
RX1  (via drill 0.61)
  Top 0.254: v130.82,21.3 129.72,20.2 v129.72,19.3 | v94.32,19 90.82,22.5 IC7.1
  Bottom 0.254: v130.82,21.3 132.82,21.3 133.42,21.9 IC5.7 | v129.72,19.3 128.12,17.7 100.32,17.7 99.02,19 v94.32,19
S88N_CLK  (via drill 0.5)
  Top 0.2: v59.81,32.7 v41.81,32.7 40.11,32.7 39.11,31.7 v34.91,31.7 | v16.41,53.2 14.91,53.2 14.41,53.7 X2.4 | v16.71,34.5 17.31,33.9 22.11,33.9 24.31,31.7 v29.11,31.7 | v41.21,43.5 41.21,44.8 U1.43
  Bottom 0.2: v59.81,32.7 62.51,35.4 62.51,41.6 64.61,43.7 64.61,45.9 65.61,46.9 X1.4 | v16.41,53.2 16.71,52.9 v16.71,34.5 | v34.91,31.7 v29.11,31.7 | v41.81,32.7 41.91,32.8 41.91,36.9 40.61,38.2 40.61,40.7 41.01,41.1 41.01,41.5 41.51,42 41.51,43.2 v41.21,43.5
S88N_PS  (via drill 0.5)
  Top 0.2: v61.51,45.6 52.31,45.6 49.01,42.3 43.51,42.3 41.71,44.1 41.71,44.81 U1.44 41.71,44.8 | v63.81,49 64.31,49.5 X1.6 | v11.61,22.3 12.41,21.5 v55.31,21.5
  Bottom 0.2: v63.81,49 63.81,47.9 v61.51,45.6 60.81,45.6 60.01,44.8 60.01,34.5 57.31,31.8 57.31,23.5 v55.31,21.5 | v11.61,22.3 11.61,27.8 13.71,29.9 13.71,36.8 13.11,37.4 13.11,49.9 14.31,51.1 X2.6
S88N_RAILDATA  (via drill 0.5)
  Top 0.2: v64.21,46.9 51.21,46.9 50.71,47.4 49.71,47.4 49.61,47.3 45.71,47.3 U1.50 | v19.11,78.7 19.21,78.6 62.01,78.6 v62.11,78.7
  Bottom 0.2: v64.21,46.9 64.61,47.3 64.61,51 65.61,52 X1.8 65.11,51.6 65.11,68.9 62.41,71.6 62.41,78.4 v62.11,78.7 | v19.11,78.7 19.11,73.3 16.81,71 16.81,54.8 15.61,53.6 15.61,49.9 14.41,48.7 X2.8
S88N_RST  (via drill 0.5)
  Top 0.2: v42.41,46.7 42.21,46.7 42.21,44.9 U1.45 | 57.51,41.5 64.11,41.5 67.21,44.6 70.31,44.6 71.41,45.7 71.41,48.7 69.41,50.7 68.21,50.7 X1.7 | 57.51,41.5 51.71,41.5 51.01,42.2 49.71,42.2 49.31,41.8 42.91,41.8 v42.71,42 | v13.91,46.6 12.17,46.6 11.91,46.85 11.91,49.9 X2.7 | 57.51,41.5 v57.51,41.4
  Bottom 0.2: v42.41,46.7 42.91,46.2 42.91,42.2 v42.71,42 | v13.91,46.6 14.11,46.4 14.11,9.2 17.41,5.9 17.41,5.6 18.21,4.8 46.91,4.8 47.91,5.8 47.91,7.9 49.61,9.6 49.61,21.1 52.21,23.7 52.21,30.2 57.51,35.5 v57.51,41.4
S88N_RX  (via drill 0.5)
  Top 0.2: v43.21,47.5 42.11,47.5 40.71,46.1 40.71,44.9 U1.42 | v64.91,40.6 50.41,40.6 50.11,40.2 49.21,40.2 48.61,40.8 44.01,40.8 43.71,40.5 v43.71,40.4
  Bottom 0.2: v43.21,47.5 43.71,47 v43.71,40.4 | v64.91,40.6 65.61,41.3 65.61,44.4 X1.2
S88N_TX  (via drill 0.5)
  Top 0.2: v24.61,32.5 v38.81,32.5 | v21.51,53.2 19.71,55 15.61,55 14.41,56.2 X2.2 | U1.41 40.19,44.02 v39.51,43.4
  Bottom 0.2: v38.81,32.5 39.11,32.8 39.11,36.8 37.91,38 37.91,42.5 38.81,43.4 v39.51,43.4 | v24.61,32.5 23.41,32.5 21.91,34 21.91,40.7 21.51,41.1 v21.51,53.2
S88N_VCC  (via drill 0.5)
  Top 0.2: v14.01,78.8 14.01,80.8 76.61,80.8 79.11,78.3 79.11,51.3 v72.01,44.2
  Bottom 0.2: X1.1 68.21,43.1 SJ3.2 70.51,43.1 v72.01,44.2 | v14.01,78.8 14.01,73.3 11.71,71 11.71,57.7 11.81,57.6 X2.1
SPI_CLK  (via drill 0.5)
  Top 0.2: v29.61,41.1 29.61,42.6 29.81,42.8 36.08,42.8 36.71,43.44 36.71,44.8 U1.34 | JP3.7 22.71,49.8 24.21,48.3 25.61,48.3 27.31,46.6 v27.91,46.6
  Bottom 0.2: v29.61,41.1 27.91,42.8 v27.91,46.6
SPI_CS  (via drill 0.5)
  Top 0.2: v26.21,45.2 34.51,45.2 34.88,44.83 U1.33
  Bottom 0.2: v26.21,45.2 26.21,48.8 25.21,49.8 JP3.8
SPI_MISO
  Top 0.2: U1.35 37.21,44.9 37.21,45.8 26.71,45.8 25.21,47.3 JP3.10
SPI_MOSI  (via drill 0.5)
  Top 0.2: v34.71,41.4 37.08,41.4 37.71,42.03 37.71,44.8 U1.36
  Bottom 0.2: v34.71,41.4 34.31,41 34.31,35.2 31.71,32.6 26.35,32.6 23.81,35.13 23.81,39.4 22.01,41.2 22.01,46.7 22.61,47.3 JP3.9
SWCLK  (via drill 0.5)
  Top 0.2: v50.41,46.6 45.81,46.6 45.71,46.7 U1.49 | v51.51,47.7 51.81,48 v58.51,48 | v60.71,67.9 60.31,67.5 45.21,67.5 44.91,67.8 41.61,67.8 40.71,66.9 40.11,66.9 39.71,67.3 5.71,67.3 v5.51,67.5
  Bottom 0.2: v51.51,47.7 v50.41,46.6 | v58.51,48 59.81,49.3 59.81,67 v60.71,67.9 | v5.51,67.5 3.51,65.5 3.51,61.4 3.21,61.1 3.21,57.6 3.51,57.3 3.51,53.5 1.91,51.9 JP36.2
SWDIO  (via drill 0.5)
  Top 0.2: v46.71,43.6 45.91,42.8 43.71,42.8 42.71,43.8 42.71,44.9 U1.46 | v20.41,32.7 20.01,33.1 v11.01,33.1 | v4.41,56.6 4.21,56.8 1.91,56.8 JP36.4
  Bottom 0.2: v46.71,43.6 46.71,32.4 43.71,29.4 21.41,29.4 20.41,30.4 v20.41,32.7 | v11.01,33.1 8.61,35.5 8.61,38.9 5.91,41.6 5.91,44.1 8.41,46.6 8.41,52.6 v4.41,56.6
TP  (via drill 0.61)
  Top 0.254: v95.02,75.7 95.02,77.1 C7.1
  Bottom 0.254: v95.02,75.7 95.02,77 95.32,77 R76.2 94.92,77 93.62,77 R77.1
TP1  (via drill 0.61)
  Top 0.254: v95.02,23.7 95.02,25.1 C17.1
  Bottom 0.254: v95.02,23.7 95.02,25 95.32,25 R86.2 94.92,25 93.62,25 R87.1
TX  (via drill 0.61)
  Top 0.254: v125.72,66.3 125.22,66.3 124.02,65.1 123.22,65.1 123.22,60.5 v123.42,60.3
  Bottom 0.254: v125.72,66.3 126.12,65.9 130.02,65.9 130.02,68 133.42,71.4 IC2.8 | v123.42,60.3 123.02,60.7 98.22,60.7 92.02,66.9 90.82,66.9 IC4.4
TX1  (via drill 0.61)
  Top 0.254: v125.72,14.3 125.22,14.3 124.02,13.1 123.22,13.1 123.22,8.5 v123.42,8.3
  Bottom 0.254: v125.72,14.3 126.12,13.9 130.02,13.9 130.02,16 133.42,19.4 IC5.8 | v123.42,8.3 123.02,8.7 98.22,8.7 92.02,14.9 90.82,14.9 IC7.4
V3_3  (via drill 0.5)
  Top 0.2: 76.61,38.3 R49.2 | v55.61,39.7 55.61,38.3 55.91,38.3 R53.2 56.01,38.2 58.11,38.2 R52.2 58.21,38.3 58.21,40 64.41,40 66.11,38.3 R51.2 66.21,38.2 68.31,38.2 R50.2 68.41,38.3 v70.11,40 71.11,40 | R47.2 R46.2 71.31,62.6 71.31,61 65.01,61 R45.2 R44.2 61.11,62.6 61.11,61 54.01,61 | R40.2 R41.2 43.11,62.7 44.01,63.6 44.01,64 44.81,64.8 44.81,66.2 44.91,66.2 45.41,66.7 47.01,66.7 | 51.01,62.7 R43.2 54.01,62.7 54.01,61 | 54.01,61 54.01,58.2 53.81,58 53.71,58 52.91,57.2 R48.2 53.11,57.3 55.21,55.2 59.91,55.2 61.51,53.6 C2.+ 61.61,53.5 69.81,53.5 71.81,51.5 71.81,45.5 71.11,44.8 71.11,40 | 47.01,66.7 48.61,66.7 49.81,65.5 49.81,63.8 49.91,63.8 51.01,62.7 | 51.01,62.7 R42.2 | 28.11,40.1 28.11,38.3 27.91,38.3 R58.2 27.81,38.2 25.71,38.2 R59.2 25.61,38.3 23.91,40 19.41,40 17.71,38.3 R60.2 17.61,38.2 15.51,38.2 R61.2 15.41,38.3 13.71,40 7.61,40 | 28.11,40.1 28.11,41.8 R64.2 | v32.91,46.8 34.21,46.8 U1.32 | R56.2 37.91,38.2 35.81,38.2 R57.2 35.71,38.3 35.51,38.3 v35.51,39.7 35.11,40.1 28.11,40.1 | R63.2 5.41,38.2 7.51,38.2 R62.2 7.61,38.3 7.61,40 | 7.61,40 5.01,42.6 1.91,42.6 1.91,49.2 JP36.1 2.01,49.2 6.71,53.9 12.21,53.9 12.91,54.6 12.91,56.5 9.41,56.5 7.51,58.4 7.51,61 | 2.41,61.1 2.41,61 2.51,61 | 2.41,61.1 2.41,62.7 R3.2 | 7.51,61 8.61,61 R4.2 | R4.2 R35.2 14.21,61 19.91,61 v20.11,61.2 20.11,62.7 R36.2 22.61,62.7 | R4.2 | R39.2 R38.2 30.61,62.7 30.61,61 24.31,61 22.61,62.7 | 22.61,62.7 R37.2 | R54.2 48.01,38.2 46.01,38.2 R55.2 46.01,38.1 44.51,36.6 v44.51,34.7 | v44.51,45 43.81,45 43.71,44.9 U1.48 | 37.71,54.1 37.71,53.7 35.81,53.7 35.41,53.3 34.31,53.3 U1.19 34.21,53.3 32.91,53.3 32.61,53.6 26.41,53.6 25.21,52.4 JP3.6
  Top 0.2: 37.71,54.1 37.71,54.9 | 37.71,54.9 37.71,56.2 U1.13 | 37.71,54.1 40.51,54.1 40.71,54.3 v44.21,54.3 45.61,54.3 U1.64 | 37.71,54.9 v37.41,54.9 | v47.01,66.3 47.01,66.7 | 7.51,61 2.51,61 | 2.51,61 2.41,61.1 | 71.11,40 73.71,40 74.01,39.7 76.41,39.7 | 76.41,39.7 76.41,38.4 76.51,38.3 | v77.11,39.7 76.41,39.7
  Bottom 0.2: IC1.2 72.41,48.2 73.71,46.9 73.71,44.8 71.31,42.4 71.31,41.6 71.21,41.5 70.11,41.5 | v77.11,39.7 77.11,43.5 78.31,44.7 C4.1 | R65.2 54.01,51.7 54.01,49.6 R66.2 55.11,48.4 55.11,47.6 56.11,46.6 SJ4.2 56.01,46.6 55.61,46.2 v55.61,39.7 | v70.11,40 70.11,41.5 | 70.11,41.5 SJ3.1 | 34.41,46.8 v32.91,46.8 | 34.41,46.8 34.41,47.2 C6.1 34.41,46.8 | 34.41,46.8 35.51,45.7 v35.51,39.7 | v20.11,61.2 20.11,60.1 R67.2 20.11,60 21.51,60 21.51,59.3 21.71,59.1 21.71,58 21.61,57.9 21.61,54.6 22.31,53.9 23.56,53.9 23.81,54.15 23.81,55 24.71,55.9 26.21,55.9 | C9.1 44.51,52.5 v44.51,45 v44.51,34.7 | 26.21,55.9 26.21,53.4 25.21,52.4 JP3.6 | v37.41,54.9 37.41,56 37.11,56.3 C5.1 | v44.21,54.3 45.21,53.3 C9.1 | v47.01,66.3 46.71,66 46.71,62.2 46.21,61.7 46.21,54.3 45.61,53.7 C9.1 | R68.2 27.81,57.5 26.21,55.9
  pour Top: 79.51,34 79.51,67 0.51,67 0.51,34
V5_0  (via drill 0.5)
  Top 0.2: v63.41,43.7 65.21,45.5 66.51,45.5 67.71,46.7 v69.71,46.7
  Bottom 0.2: C3.1 71.51,54 71.51,51.35 IC1.3 | 72.31,50.6 IC1.3 | 69.81,46.7 69.81,48 72.31,50.5 IC1.3 | 69.81,46.7 69.81,45 70.11,44.7 SJ3.3 | v63.41,43.7 61.71,43.7 C1.+ | 69.81,46.7 v69.71,46.7
VDD  (via drill 0.61)
  Top 0.508: v145.22,68.8 144.52,69.5 144.52,71.3 C12.+ 144.52,71.6 144.82,71.9 144.82,76.9 145.32,77.4 IC3.OUT 145.32,77.7 144.22,78.8 144.22,90.2 v144.02,90.4 | v127.32,80 127.32,78.9 | 127.32,78.9 127.32,76.9 | 127.32,76.9 127.32,72.4 v127.22,72.3 127.32,72.1 127.32,61.7 v127.62,61.4 | v126.32,84.1 125.32,83.1 125.32,80.7 127.12,78.9 127.32,78.9 | v122.12,82 123.02,81.1 123.02,77.7 123.82,76.9 127.32,76.9
  Bottom 0.508: R73.2 152.22,97.1 148.62,97.1 JP37.2 148.42,97.3 147.32,98.4 142.12,98.4 141.62,97.9 141.62,90.4 v144.02,90.4 | 144.42,77.4 144.42,75.3 C15.1 | 144.42,77.4 145.32,77.4 IC3.OUT | v145.22,68.8 154.02,68.8 154.02,64.5 155.52,63 155.62,63 JP39.2 | IC4.8 98.42,74.6 94.62,74.6 93.42,75.8 89.52,75.8 89.52,77.6 R78.1 95.82,83.6 97.42,82 v122.12,82 | 128.67,81.35 128.92,81.1 131.52,81.1 132.42,80.2 137.02,80.2 138.02,79.2 C16.1 138.12,79 141.02,79 IC2.14 141.32,79 142.72,79 144.22,77.5 144.42,77.4 | 128.67,81.35 127.72,82.3 R70.2 | v127.22,72.3 127.62,72.3 127.62,71 R71.2 | 128.67,81.35 v127.32,80 | v127.62,61.4 127.62,60 R72.2 | v126.32,84.1 126.82,84.1 126.82,86.8 R69.2
  pour Bottom: 159.02,53.5 88.52,53.5 88.52,99.5 159.02,99.5
VDD1  (via drill 0.61)
  Top 0.508: v145.22,16.8 144.52,17.5 144.52,19.3 C20.+ 144.52,19.6 144.82,19.9 144.82,24.9 145.32,25.4 IC6.OUT 145.32,25.7 144.22,26.8 144.22,38.2 v144.02,38.4 | v127.32,28 127.32,26.9 | 127.32,26.9 127.32,24.9 | 127.32,24.9 127.32,20.4 v127.22,20.3 127.32,20.1 127.32,9.7 v127.62,9.4 | v126.32,32.1 125.32,31.1 125.32,28.7 127.12,26.9 127.32,26.9 | v122.12,30 123.02,29.1 123.02,25.7 123.82,24.9 127.32,24.9
  Bottom 0.508: R83.2 152.22,45.1 148.62,45.1 JP40.2 148.42,45.3 147.32,46.4 142.12,46.4 141.62,45.9 141.62,38.4 v144.02,38.4 | 144.42,25.4 144.42,23.3 C23.1 | 144.42,25.4 145.32,25.4 IC6.OUT | v145.22,16.8 154.02,16.8 154.02,12.5 155.52,11 155.62,11 JP42.2 | IC7.8 98.42,22.6 94.62,22.6 93.42,23.8 89.52,23.8 89.52,25.6 R88.1 95.82,31.6 97.42,30 v122.12,30 | 128.67,29.35 128.92,29.1 131.52,29.1 132.42,28.2 137.02,28.2 138.02,27.2 C24.1 138.12,27 141.02,27 IC5.14 141.32,27 142.72,27 144.22,25.5 144.42,25.4 | 128.67,29.35 127.72,30.3 R80.2 | v127.22,20.3 127.62,20.3 127.62,19 R81.2 | 128.67,29.35 v127.32,28 | v127.62,9.4 127.62,8 R82.2 | v126.32,32.1 126.82,32.1 126.82,34.8 R79.2
  pour Bottom: 159.02,1.5 88.52,1.5 88.52,47.5 159.02,47.5
VIN  (via drill 0.61)
  Top 0.508: v151.02,79.4 151.02,80.8 152.22,82 C11.+
  Bottom 0.508: 148.92,77.4 C14.1 149.02,75 150.22,75 150.22,71.3 D133.C | 148.92,77.4 147.92,77.4 IC3.IN | v151.02,79.4 149.12,77.5 148.92,77.4
VIN1  (via drill 0.61)
  Top 0.508: v151.02,27.4 151.02,28.8 152.22,30 C19.+
  Bottom 0.508: 148.92,25.4 C22.1 149.02,23 150.22,23 150.22,19.3 D138.C | 148.92,25.4 147.92,25.4 IC6.IN | v151.02,27.4 149.12,25.5 148.92,25.4
VO
  Top 0.254: 154.92,64.1 156.82,64.1 JP39.3 | 154.92,64.1 153.12,64.1 R74.2 | 154.92,64.1 154.92,92.5 149.12,98.3 147.22,98.3 147.22,96.4 146.12,95.3 146.12,94.6 JP37.3
  Bottom 0.254: R73.1 152.22,95.5 152.02,95.7 147.22,95.7 146.12,94.6 JP37.3
VO1
  Top 0.254: 154.92,12.1 156.82,12.1 JP42.3 | 154.92,12.1 153.12,12.1 R84.2 | 154.92,12.1 154.92,40.5 149.12,46.3 147.22,46.3 147.22,44.4 146.12,43.3 146.12,42.6 JP40.3
  Bottom 0.254: R83.1 152.22,43.5 152.02,43.7 147.22,43.7 146.12,42.6 JP40.3
XVDD
  Bottom 0.508: D133.A 144.12,70.2 144.12,67.4 144.52,67.4 J1.5
XVDD1
  Bottom 0.508: D138.A 144.12,18.2 144.12,15.4 144.52,15.4 J2.5

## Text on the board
Top: 1 | 2012 | mmv2 | 2012 | mmv2
Bottom: AWA | 2012 | 1 | GBM32ST V1.0 | AWA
